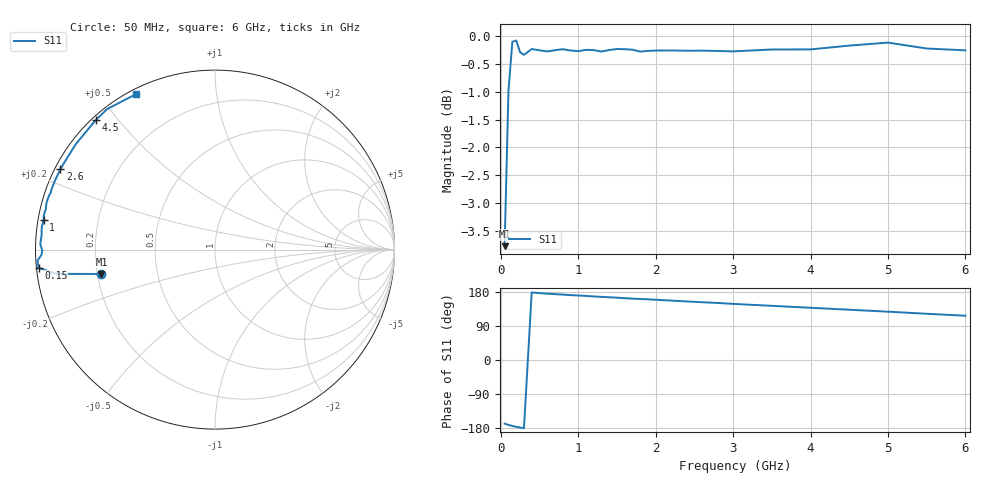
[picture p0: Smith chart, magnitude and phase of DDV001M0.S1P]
! Infineon Technologies  Discrete & RF Semiconductors
! BBY58-02W
! Si Tuning Diode in SCD-80
! VR =
! S-Parameters:  June  2000
# GHz  S  MA  R  50
!  f  S11
! GHz  MAG  ANG
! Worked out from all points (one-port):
!   34 points, 50 MHz to 6 GHz, reference 50 ohm
!   lowest |S11| = -3.8 dB at 50 MHz (marker M1), VSWR 4.67, Z = 10.8 - j5.05 ohm
!   |S11| at or under -10 dB: nowhere
!   S11 on the Smith chart (normalised r, x): 50 MHz: 0.22, -0.10; 150 MHz: 0.01, -0.05; 1 GHz: 0.02, +0.09; 2.6 GHz: 0.02, +0.24; 4.5 GHz: 0.01, +0.44; 6 GHz: 0.02, +0.62
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0.05  0.6473 -167.9
0.1  0.8933 -171.3
0.15  0.9885 -174.1
0.2  0.9913 -176.4
0.25  0.9673 -178.3
0.3  0.9622 -179.7
0.4  0.9738 178.2
0.6  0.969 175.1
0.8  0.9735 172.6
1  0.9695 170.2
1.1  0.9722 169.1
1.2  0.9717 167.7
1.3  0.9688 166.6
1.5  0.9739 164.5
1.6  0.9735 163.2
1.7  0.9726 162.0
1.8  0.9686 161.0
1.9  0.9701 160.2
2.4  0.9704 154.5
2.6  0.9706 152.5
2.8  0.97 150.5
3  0.9691 148.1
3.5  0.9729 143.0
4  0.9731 137.8
4.5  0.9808 132.7
5  0.9869 127.5
5.5  0.9749 122.0
6  0.9712 116.8
